(* Logix 5000 DataType export AMCI_Motion_Axis_Input_Data; software revision 20.03 *)

TYPE AMCI_Motion_Axis_Input_Data :
STRUCT
   Moving_CW : BOOL;
   Moving_CCW : BOOL;
   In_Hold_State : BOOL;
   Stopped : BOOL;
   At_Home : BOOL;
   Accelerating : BOOL;
   Decelerating : BOOL;
   Move_Complete : BOOL;
   Status_Word_0_Bit_8 : BOOL;
   Status_Word_0_Bit_9 : BOOL;
   Position_Invalid : BOOL;
   Input_Error : BOOL;
   Command_Error : BOOL;
   Configuration_Error : BOOL;
   Module_OK : BOOL;
   Mode_Flag : BOOL;
   IN1_Active : BOOL;
   IN2_Active : BOOL;
   IN3_Active : BOOL;
   IN4_Active : BOOL;
   Status_Word_1_Bit_4 : BOOL;
   Status_Word_1_Bit_5 : BOOL;
   Connection_Was_Lost : BOOL;
   Driver_Fault : BOOL;
   Status_Word_1_Bit_8 : BOOL;
   Invalid_Jog_Change : BOOL;
   Status_Word_1_Bit_10 : BOOL;
   Heartbeat_Bit : BOOL;
   Status_Word_1_Bit_12 : BOOL;
   Status_Word_1_Bit_13 : BOOL;
   Stall_Detected : BOOL;
   Drive_Is_Enabled : BOOL;
   Motor_Position : DINT;
   Encoder_Position : DINT;
   Trapped_Encoder_Position : DINT;
   Input_Word_8 : INT;
   Input_Word_9 : INT;
END_STRUCT
END_TYPE
